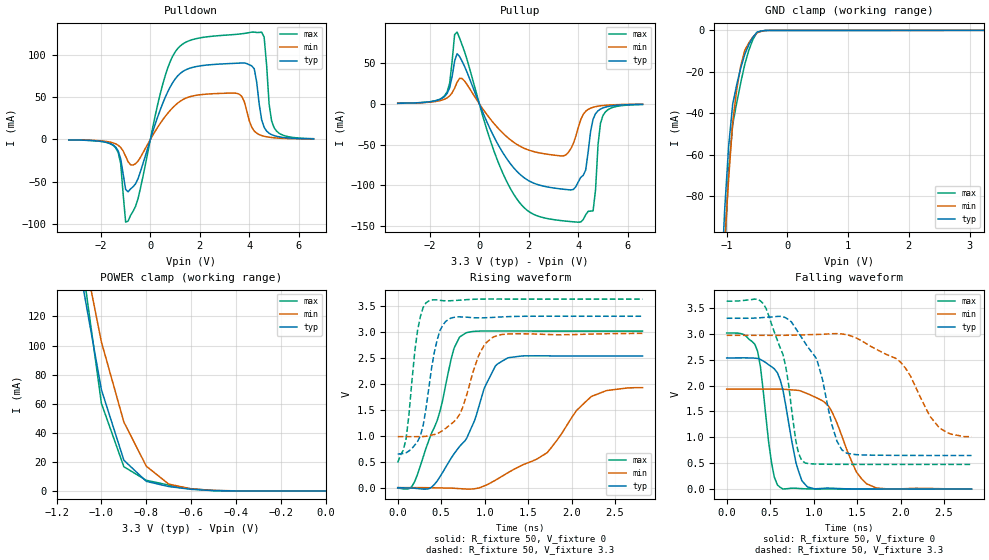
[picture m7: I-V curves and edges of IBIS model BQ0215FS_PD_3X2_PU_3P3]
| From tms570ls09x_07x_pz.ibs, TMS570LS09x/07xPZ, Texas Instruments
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|   Model Cell BQ0215FS_PD_3X2_PU_3P3
|BQ0215FS_PD_3X2_PU_3P3
[Model]   BQ0215FS_PD_3X2_PU_3P3
Model_type   I/O
Polarity   Non-Inverting
Enable   Active-Low
Vinl =  1.25
Vinh =  1.65
Cref =  15.0001pF
Rref =  101.0000M
Vref =  0V
Vmeas =  1.65
C_comp   1.2p   1.2p   1.2p
[Model Spec]
Vinl   1.25   1.12   1.38
Vinh   1.65   1.45   1.75
[Temperature Range]   25   155   -40
[Voltage Range]   3.3   2.97   3.63
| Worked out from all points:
|   slope of the pulldown table from 0 to 0.495 V, typ, clamps not added: 11.8 ohm
|   slope of the pullup table from 0 to 0.495 V, typ, clamps not added: 14.3 ohm
|   GND clamp passes 1 mA (typ) near -0.50 V on its own axis
|   POWER clamp passes 1 mA (typ) near -0.59 V on its own axis
|   rising waveform, R_fixture 50, V_fixture 0: 20-80 % time 436ps typ, 716ps min, 312ps max; typ from 0 V to 2.53 V
|   rising waveform, R_fixture 50, V_fixture 3.3: 20-80 % time 154ps typ, 240ps min, 117ps max; typ from 0.649 V to 3.3 V
|   falling waveform, R_fixture 50, V_fixture 0: 20-80 % time 169ps typ, 283ps min, 125ps max; typ from 2.53 V to 0 V
|   falling waveform, R_fixture 50, V_fixture 3.3: 20-80 % time 299ps typ, 472ps min, 225ps max; typ from 3.3 V to 0.648 V
[POWER_clamp]
|   voltage   I(typ)   I(min)   I(max)
-3.3V     2.375A     2.63A      3.153A
-1.1V     156mA      180.2mA    173.4mA
-1.067V   127.2mA    154.3mA    135.7mA
-1.033V   98.42mA    128.4mA    97.93mA
-1V       69.62mA    102.5mA    60.21mA
-900mV    21.14mA    47.42mA    16.63mA
-800mV    6.589mA    17.01mA    7.329mA
-700mV    3.011mA    4.694mA    4.008mA
-600mV    1.098mA    1.411mA    1.442mA
-500mV    196.6uA    363.8uA    217.1uA
0V        429.9pA    12.78nA    319.2pA
[Pulldown]
|   voltage   I(typ)   I(min)   I(max)
-3.3V     -560.7uA   -504.5uA   -563.6uA
-1.4V     -9.199mA   -5.273mA   -10.11mA
-1.2V     -22.91mA   -9.491mA   -28.67mA
-1V       -59mA      -19.85mA   -97.49mA
-900mV    -61.64mA   -26.24mA   -96.13mA
1V        71.11mA    40.13mA    102.9mA
3.5V      89.74mA    54.24mA    123.8mA
4.2V      83.16mA    9.923mA    126.4mA
4.6V      14.26mA    3.714mA    120.5mA
4.8V      7.317mA    2.617mA    42.02mA
5V        4.531mA    1.939mA    13.99mA
6.6V      631.1uA    487.2uA    853.6uA
[Pullup]
|   voltage   I(typ)   I(min)   I(max)
-3.3V     614.6uA    591.9uA    551.1uA
-1.4V     9.028mA    5.738mA    10.01mA
-900mV    61.32mA    26.24mA    87.8mA
500mV     -34.85mA   -20.79mA   -49.88mA
1.4V      -78.76mA   -47.33mA   -111.2mA
3.4V      -104.6mA   -63.81mA   -143.4mA
4V        -95.71mA   -29.08mA   -145mA
4.3V      -81.25mA   -9.188mA   -136.1mA
4.6V      -18.8mA    -4.29mA    -131.2mA
4.8V      -8.576mA   -2.945mA   -49.93mA
5V        -5.064mA   -2.148mA   -14.33mA
6.6V      -672.1uA   -541.9uA   -866.9uA
[GND_clamp]
|   voltage   I(typ)   I(min)   I(max)
-3.3V     -1.951A    -1.627A    -3.261A
-1.1V     -130.1mA   -138.8mA   -166.7mA
-1.033V   -87.46mA   -103.2mA   -108mA
-966.7mV  -55.98mA   -71.78mA   -67.59mA
-900mV    -35.71mA   -44.42mA   -45.59mA
-833.3mV  -26.16mA   -28.61mA   -34.93mA
-766.7mV  -18.1mA    -17.01mA   -25.16mA
-700mV    -11.52mA   -9.614mA   -16.29mA
-633.3mV  -6.852mA   -5.986mA   -9.523mA
-500mV    -890.3uA   -1.251mA   -1.035mA
-300mV    -21.3uA    -25.97uA   -33.69uA
3.233V    -1.13uA    6.932uA    -9.303uA
[Ramp]
| variable   typ   min   max
dV/dt_f   1.614145/0.3078799n   1.213428/0.5100454n   1.917729/0.231895n
dV/dt_r   1.540834/0.443378n   1.175982/0.7399471n   1.826864/0.314532n
R_load = 50
[Rising Waveform]
R_fixture = 50
V_fixture = 0
V_fixture_min = 0
V_fixture_max = 0
|   time   V(typ)   V(min)   V(max)
0s        71.21uV    232.4uV    -8.133mV
196ps     -11.38mV   461.3uV    119.9mV
484ps     205.3mV    -4.893mV   1.457V
648ps     652.1mV    -11.43mV   2.685V
776ps     907.3mV    -24.97mV   2.97V
1.124ns   2.344V     143.7mV    3.016V
1.268ns   2.5V       288.1mV    3.015V
1.72ns    2.537V     675mV      3.014V
2.228ns   2.534V     1.756V     3.014V
2.816ns   2.534V     1.925V     3.014V
[Rising Waveform]
R_fixture = 50
V_fixture = 3.3
V_fixture_min = 2.97
V_fixture_max = 3.63
|   time   V(typ)   V(min)   V(max)
0s        648.6mV    982.5mV    482.2mV
96ps      672mV      981.8mV    939.7mV
228ps     889.3mV    982.1mV    3.028V
324ps     1.508V     988.2mV    3.557V
452ps     2.832V     1.035V     3.615V
616ps     3.267V     1.228V     3.599V
744ps     3.287V     1.53V      3.613V
952ps     3.269V     2.616V     3.63V
1.104ns   3.279V     2.904V     3.631V
2.816ns   3.3V       2.969V     3.63V
[Falling Waveform]
R_fixture = 50
V_fixture = 0
V_fixture_min = 0
V_fixture_max = 0
|   time   V(typ)   V(min)   V(max)
0s        2.534V     1.93V      3.015V
356ps     2.523V     1.93V      2.659V
516ps     2.364V     1.931V     510.2mV
616ps     2.107V     1.931V     32.85mV
796ps     513.8mV    1.91V      15.13mV
928ps     42.04mV    1.843V     3.085mV
1.192ns   17.21mV    1.549V     255.7uV
1.492ns   1.603mV    328.4mV    222.2uV
1.608ns   740.3uV    102.4mV    202.3uV
2.816ns   261.1uV    1.518mV    185uV
[Falling Waveform]
R_fixture = 50
V_fixture = 3.3
V_fixture_min = 2.97
V_fixture_max = 3.63
|   time   V(typ)   V(min)   V(max)
0s        3.3V       2.97V      3.63V
452ps     3.319V     2.97V      3.492V
648ps     3.329V     2.97V      2.6V
796ps     3.098V     2.974V     926.7mV
884ps     2.869V     2.978V     526.3mV
1.036ns   2.508V     2.987V     482.8mV
1.38ns    692.9mV    2.982V     476.5mV
2ns       650.1mV    2.453V     475.7mV
2.46ns    648.5mV    1.165V     475.8mV
2.816ns   648.3mV    1.013V     475.9mV
